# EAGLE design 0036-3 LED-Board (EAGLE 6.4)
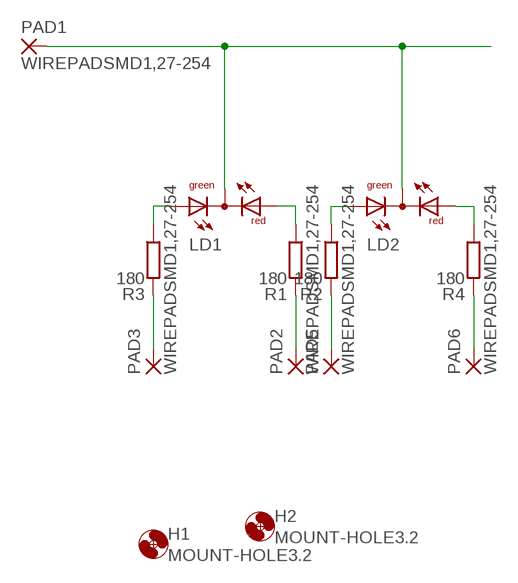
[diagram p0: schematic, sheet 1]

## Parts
H1  MOUNT-HOLE3.2  [3,2]
H2  MOUNT-HOLE3.2  [3,2]
LD1  DUOLED-RG-C  [DUOLED-C-5MM]
LD2  DUOLED-RG-C  [DUOLED-C-5MM]
PAD1  WIREPADSMD1,27-254  [SMD1,27-2,54]
PAD2  WIREPADSMD1,27-254  [SMD1,27-2,54]
PAD3  WIREPADSMD1,27-254  [SMD1,27-2,54]
PAD5  WIREPADSMD1,27-254  [SMD1,27-2,54]
PAD6  WIREPADSMD1,27-254  [SMD1,27-2,54]
R1  180  R-EU_R0805  [R0805]
R2  180  R-EU_R0805  [R0805]
R3  180  R-EU_R0805  [R0805]
R4  180  R-EU_R0805  [R0805]

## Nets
N$1: LD1.C LD2.C PAD1.1(P)
N$2: LD1.AX(AG) R3.1
N$3: LD1.AR R1.1
N$4: LD2.AX(AG) R2.1
N$5: LD2.AR R4.1
N$6: PAD3.1(P) R3.2
N$7: PAD2.1(P) R1.2
N$8: PAD5.1(P) R2.2
N$9: PAD6.1(P) R4.2

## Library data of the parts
H1 H2 = holes:MOUNT-HOLE: MOUNTING HOLE with drill center marker
LD1 LD2 = led:DUOLED-RG-C: DUO LED 2 colors (red/green), 5 mm, round, common Cathode www.ligitek.com or other producers.
PAD1-PAD3 PAD5 PAD6 = wirepad:WIREPAD: Wire PAD connect wire on PCB
R1-R4 = rcl:R-EU_: RESISTOR, European symbol

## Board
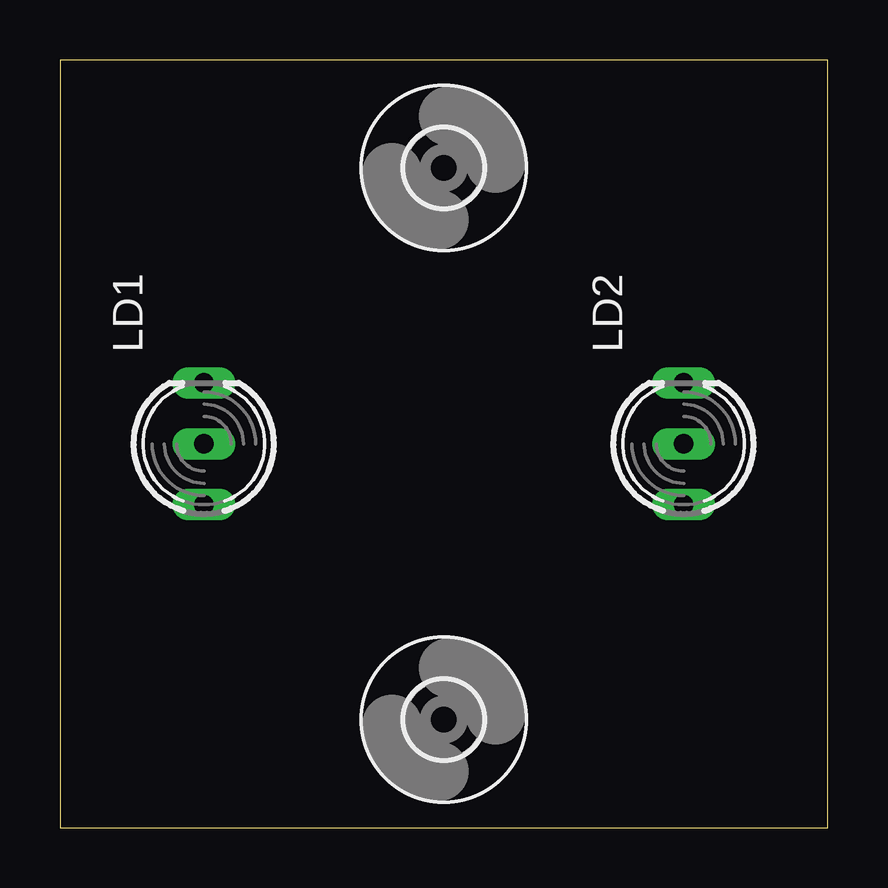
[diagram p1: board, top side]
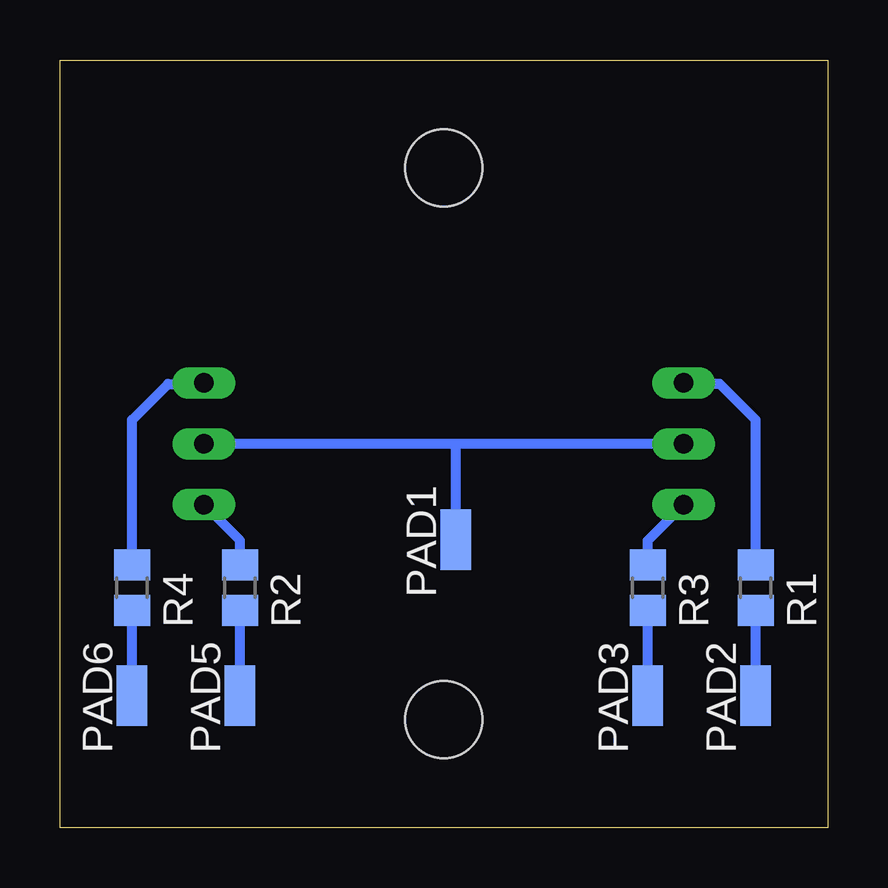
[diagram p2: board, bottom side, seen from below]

Size 32 x 32 mm. Coordinates in mm from the lower left corner, seen from the top.
Outline: 0,0 32,0 32,32 0,32 0,0
Copper layers (1*16): Top 0.035mm / dielectric 1.5mm / Bottom 0.035mm
Design rules "default": minimum track width 10mil, minimum drill 24mil, track to track 8mil, track to pad 8mil, pad to pad 8mil, via to via 8mil, smd to smd 8mil, copper to edge 40mil, drill to drill 8mil, minimum pad ring 10mil, minimum via ring 8mil, stop-mask expansion 4mil, vias tented up to drill 0mil, thermal gap 10mil

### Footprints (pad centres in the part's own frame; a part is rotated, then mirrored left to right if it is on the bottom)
3,2 = hole 3.2: 0,0
DUOLED-C-5MM = drill 0.813 long: AR 2.54,0; AX -2.54,0; C 0,0
SMD1,27-2,54 = smd 1.27 x 2.54: 1 0,0
R0805 = smd 1.3 x 1.5: 1 -0.95,0; 2 0.95,0

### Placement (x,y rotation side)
H1  16,27.5 0 top
H2  16,4.5 0 top
LD1  6,16 90 top
LD2  26,16 90 top
PAD1  15.5,12 0 bottom
PAD2  3,5.5 0 bottom
PAD3  7.5,5.5 0 bottom
PAD5  24.5,5.5 0 bottom
PAD6  29,5.5 0 bottom
R1  3,10 270 bottom
R2  24.5,10 270 bottom
R3  7.5,10 270 bottom
R4  29,10 270 bottom

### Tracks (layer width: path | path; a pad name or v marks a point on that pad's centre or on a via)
N$1
  Bottom 0.406: LD1.C 15.5,16 | 15.5,16 LD2.C | PAD1.1 15.5,16
N$2
  Bottom 0.406: R3.1 7.5,11.96 LD1.AX
N$3
  Bottom 0.406: R1.1 3,17 4.5,18.5 5.96,18.5 LD1.AR
N$4
  Bottom 0.406: R2.1 24.5,11.96 LD2.AX
N$5
  Bottom 0.406: R4.1 29,17 27.5,18.5 26.04,18.5 LD2.AR
N$6
  Bottom 0.406: PAD3.1 R3.2
N$7
  Bottom 0.406: PAD2.1 R1.2
N$8
  Bottom 0.406: PAD5.1 R2.2
N$9
  Bottom 0.406: PAD6.1 R4.2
